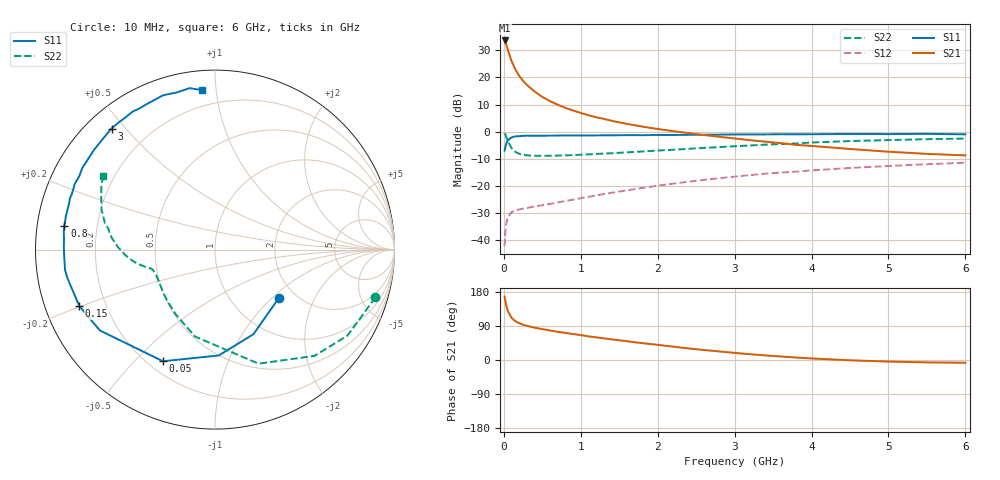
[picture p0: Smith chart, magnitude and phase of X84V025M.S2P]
! SIEMENS Small Signal Semiconductors
! BFP136W
! Si NPN RF Bipolar Junction Transistor in SOT343
! VCE = 4 V  IC = 25 mA
! Common Emitter S-Parameters:  September  1994
# GHz  S  MA  R  50
!  f  S11  S21  S12  S22
! GHz  MAG  ANG  MAG  ANG  MAG  ANG  MAG  ANG
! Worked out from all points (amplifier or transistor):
!   40 points, 10 MHz to 6 GHz, reference 50 ohm
!   highest |S21| = 33.7 dB at 10 MHz (marker M1)
!   |S21| within 3 dB of that: start of sweep to 46.75 MHz
!   unconditionally stable (mu >= 1): 844.8 MHz to 2.817 GHz
!   at 200 MHz: K = 0.38, MSG = 24.6 dB, |S12| = -28.7 dB
!   at 1.5 GHz: K = 1.14, MAG = 10.5 dB, |S12| = -22.1 dB
!   at 6 GHz: K = 0.98, MSG = 1.3 dB, |S12| = -11.4 dB
!   S11 on the Smith chart (normalised r, x): 10 MHz: 1.64, -1.11; 50 MHz: 0.26, -0.61; 150 MHz: 0.10, -0.20; 800 MHz: 0.08, +0.08; 3 GHz: 0.07, +0.46; 6 GHz: 0.11, +0.92
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0.01  0.4465 -37.1  48.17 167.2  0.0077 76.3  0.9324 -16.6
0.02  0.5178 -65.6  44.68 155.2  0.0143 66.8  0.8801 -33.0
0.03  0.5903 -88.0  41.11 145.3  0.0195 58.6  0.8109 -46.9
0.05  0.6862 -115.0  32.89 130.2  0.0263 45.0  0.6803 -69.1
0.1  0.7838 -144.9  20.12 111.4  0.0327 31.6  0.4971 -102.9
0.15  0.8189 -157.5  14.08 102.4  0.035 27.9  0.4222 -121.2
0.2  0.8251 -164.1  10.69 97.0  0.0369 26.8  0.3907 -132.7
0.25  0.8373 -169.0  8.662 93.1  0.0379 27.1  0.3755 -140.3
0.3  0.8432 -172.3  7.262 90.1  0.0389 27.4  0.3656 -145.5
0.4  0.841 -177.6  5.482 85.3  0.0417 30.4  0.3588 -152.3
0.5  0.8425 178.9  4.382 81.3  0.0438 33.3  0.3576 -156.6
0.6  0.8432 176.1  3.651 77.9  0.0463 35.7  0.3588 -159.0
0.7  0.8486 173.1  3.144 74.4  0.0493 39.1  0.3617 -160.7
0.8  0.8497 171.1  2.749 71.5  0.0526 41.0  0.3651 -161.9
1.1  0.8515 164.3  2.006 62.3  0.0626 46.2  0.381 -164.4
1.5  0.8578 157.1  1.482 52.1  0.0784 50.6  0.4069 -166.8
2.2  0.8684 144.5  1.021 35.3  0.1095 51.8  0.4635 -172.3
3  0.8872 130.5  0.748 18.8  0.1481 48.1  0.5379 178.9
3.2  0.8885 127.2  0.695 15.2  0.1574 46.6  0.5554 176.5
4.5  0.9071 108.6  0.479 -0.8  0.2134 35.6  0.6706 160.5
5.5  0.9105 99.0  0.389 -6.3  0.2501 27.5  0.7262 150.7
6  0.8922 94.7  0.365 -7.2  0.2679 23.0  0.7455 146.6
